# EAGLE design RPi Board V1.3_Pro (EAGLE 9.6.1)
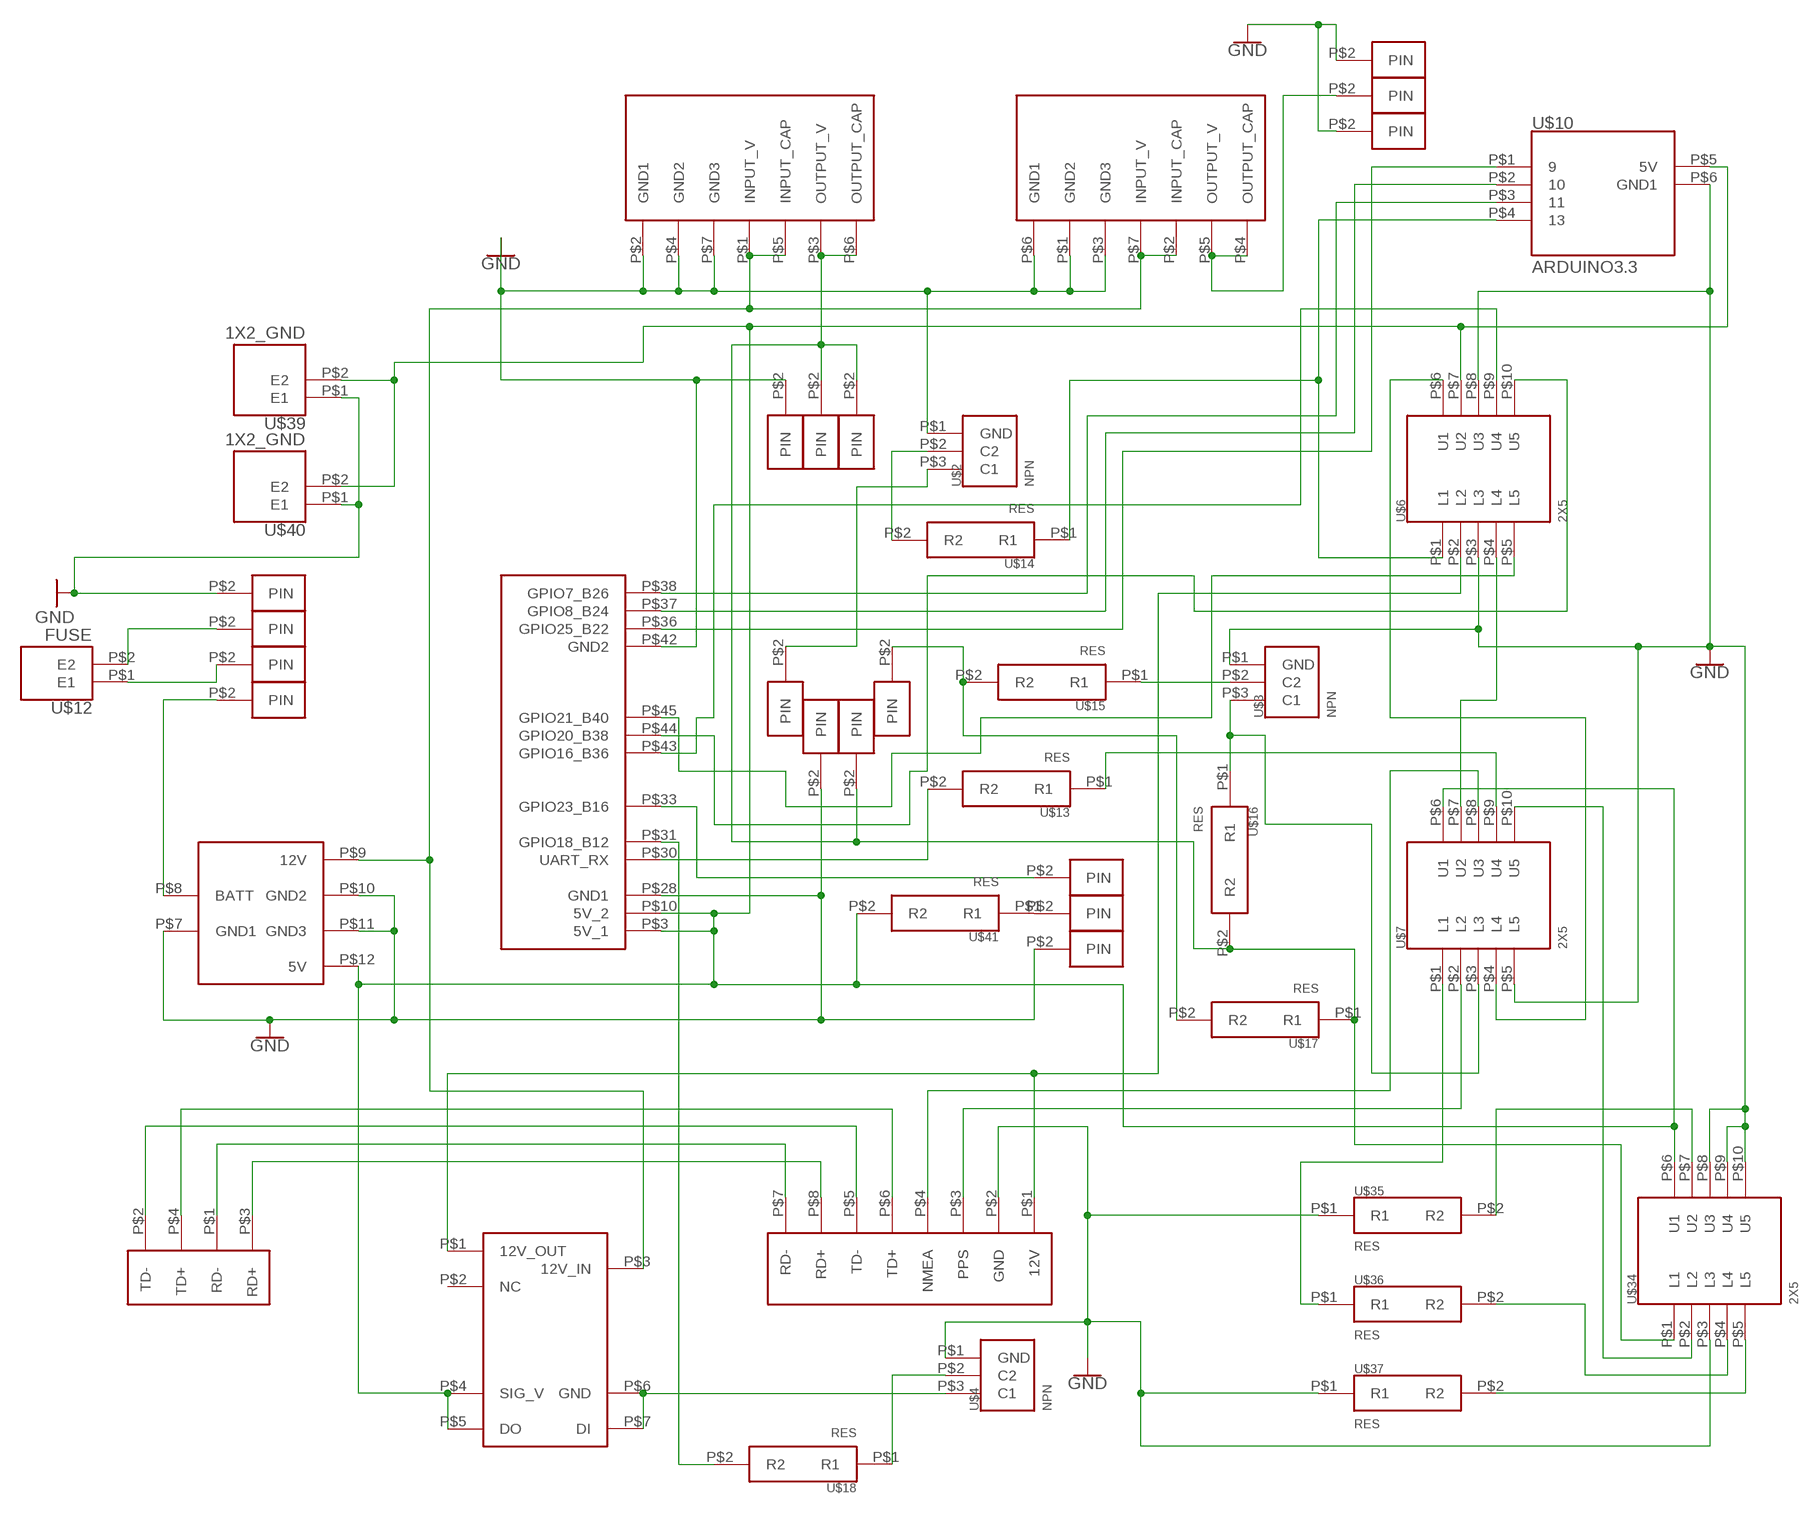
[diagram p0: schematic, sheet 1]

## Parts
U$1  RPI_1X20  [F_RPI_1X20]
U$2  NPN  [F_NPN]
U$3  NPN  [F_NPN]
U$4  NPN  [F_NPN]
U$5  LIDAR  [F_LIDAR]
U$6  2X5  [F_2X5]
U$7  2X5  [F_2X5]
U$8  3.3V_REG  [F_3.3V_REG]
U$9  9V_REG  [F_9V_REG]
U$10  ARDUINO3.3  [F_ARDUINO3.3]
U$11  ETH  [F_ETH]
U$12  FUSE  [F_FUSE]
U$13  RES  [F_RES]
U$14  RES  [F_RES]
U$15  RES  [F_RES]
U$16  RES  [F_RES]
U$17  RES  [F_RES]
U$18  RES  [F_RES]
U$19  1X1  [F_1X1]
U$20  1X1  [F_1X1]
U$21  1X1  [F_1X1]
U$22  1X1  [F_1X1]
U$23  12V_5V_REG  [F_12V_5V_REG]
U$24  1X1  [F_1X1]
U$25  RELAY  [F_RELAY]
U$26  1X1  [F_1X1]
U$27  1X1  [F_1X1]
U$28  1X1  [F_1X1]
U$29  1X1  [F_1X1]
U$30  1X1  [F_1X1]
U$31  1X1  [F_1X1]
U$32  1X1  [F_1X1]
U$33  1X1  [F_1X1]
U$34  2X5  [F_2X5]
U$35  RES  [F_RES]
U$36  RES  [F_RES]
U$37  RES  [F_RES]
U$38  1X1  [F_1X1]
U$39  1X2_GND  [F_1X2_GND]
U$40  1X2_GND  [F_1X2_GND]
U$41  RES  [F_RES]
U$42  1X1  [F_1X1]
U$43  1X1  [F_1X1]
U$44  1X1  [F_1X1]

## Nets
GND: U$1.P$28(GND1) U$1.P$42(GND2) U$2.P$1(GND) U$3.P$1(GND) U$4.P$1(GND) U$5.P$2(GND) U$6.P$3(L3) U$6.P$8(U3) U$7.P$5(L5) U$8.P$2(GND1) U$8.P$4(GND2) U$8.P$7(GND3) U$9.P$1(GND2) U$9.P$3(GND3) U$9.P$6(GND1) U$10.P$6(GND1) U$22.P$2(PIN) U$23.P$7(GND1) U$23.P$10(GND2) U$23.P$11(GND3) U$26.P$2(PIN) U$28.P$2(PIN) U$30.P$2(PIN) U$34.P$3(L3) U$34.P$8(U3) U$34.P$9(U4) U$34.P$10(U5) U$35.P$1(R1) U$37.P$1(R1) U$39.P$1(E1) U$40.P$1(E1) U$43.P$2(PIN) U$44.P$2(PIN)
N$1: U$12.P$2(E2) U$19.P$2(PIN)
N$2: U$12.P$1(E1) U$20.P$2(PIN)
N$3: U$21.P$2(PIN) U$23.P$8(BATT)
N$4: U$5.P$7(RD-) U$11.P$1(RD-)
N$5: U$5.P$8(RD+) U$11.P$3(RD+)
N$6: U$5.P$5(TD-) U$11.P$2(TD-)
N$7: U$41.P$1(R1) U$42.P$2(PIN)
N$8: U$8.P$3(OUTPUT_V) U$8.P$6(OUTPUT_CAP) U$16.P$2(R2) U$17.P$1(R1) U$24.P$2(PIN) U$27.P$2(PIN) U$32.P$2(PIN) U$34.P$1(L1)
N$9: U$5.P$6(TD+) U$11.P$4(TD+)
N$10: U$5.P$3(PPS) U$7.P$2(L2)
N$11: U$7.P$9(U4) U$13.P$1(R1)
N$12: U$1.P$30(UART_RX) U$13.P$2(R2)
N$13: U$5.P$1(12V) U$6.P$2(L2) U$25.P$1(12V_OUT)
N$14: U$6.P$6(U1) U$7.P$4(L4)
N$15: U$6.P$4(L4) U$7.P$7(U2)
N$16: U$1.P$3(5V_1) U$1.P$10(5V_2) U$6.P$7(U2) U$7.P$6(U1) U$10.P$5(5V) U$23.P$12(5V) U$25.P$4(SIG_V) U$25.P$5(DO) U$34.P$6(U1) U$39.P$2(E2) U$40.P$2(E2) U$41.P$2(R2)
N$17: U$5.P$4(NMEA) U$7.P$8(U3)
N$19: U$1.P$36(GPIO25_B22) U$10.P$1
N$20: U$1.P$37(GPIO8_B24) U$10.P$2
N$21: U$8.P$1(INPUT_V) U$8.P$5(INPUT_CAP) U$9.P$2(INPUT_CAP) U$9.P$7(INPUT_V) U$23.P$9(12V) U$25.P$3(12V_IN)
N$22: U$1.P$38(GPIO7_B26) U$10.P$3
N$23: U$9.P$4(OUTPUT_CAP) U$9.P$5(OUTPUT_V) U$29.P$2(PIN)
N$24: U$2.P$2(C2) U$14.P$2(R2)
N$25: U$6.P$1(L1) U$10.P$4 U$14.P$1(R1)
N$26: U$2.P$3(C1) U$31.P$2(PIN)
N$27: U$15.P$2(R2) U$17.P$2(R2) U$33.P$2(PIN)
N$28: U$3.P$2(C2) U$15.P$1(R1)
N$29: U$3.P$3(C1) U$7.P$3(L3) U$16.P$1(R1)
N$30: U$4.P$3(C1) U$25.P$6(GND) U$25.P$7(DI)
N$31: U$4.P$2(C2) U$18.P$1(R1)
N$32: U$1.P$44(GPIO20_B38) U$6.P$10(U5)
N$33: U$1.P$31(GPIO18_B12) U$18.P$2(R2)
N$34: U$1.P$43(GPIO16_B36) U$6.P$9(U4)
N$35: U$7.P$10(U5) U$34.P$2(L2)
N$36: U$34.P$7(U2) U$35.P$2(R2)
N$37: U$1.P$33(GPIO23_B16) U$38.P$2(PIN)
N$38: U$34.P$5(L5) U$37.P$2(R2)
N$39: U$34.P$4(L4) U$36.P$2(R2)
N$40: U$7.P$1(L1) U$36.P$1(R1)
N$42: U$1.P$45(GPIO21_B40) U$6.P$5(L5)
Unconnected: U$25.P$2(NC)

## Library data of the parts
U$1 = OpenMMS_Production:RPI_1X20
U$2-U$4 = OpenMMS_Production:NPN
U$5 = OpenMMS_Production:LIDAR
U$6 U$7 U$34 = OpenMMS_Production:2X5
U$8 = OpenMMS_Production:3.3V_REG
U$9 = OpenMMS_Production:9V_REG
U$10 = OpenMMS_Production:ARDUINO3.3
U$11 = OpenMMS_Production:ETH
U$12 = OpenMMS_Production:FUSE
U$13-U$18 U$35-U$37 U$41 = OpenMMS_Production:RES
U$19-U$22 U$24 U$26-U$33 U$38 U$42-U$44 = OpenMMS_Production:1X1
U$23 = OpenMMS_Production:12V_5V_REG
U$25 = OpenMMS_Production:RELAY
U$39 U$40 = OpenMMS_Production:1X2_GND

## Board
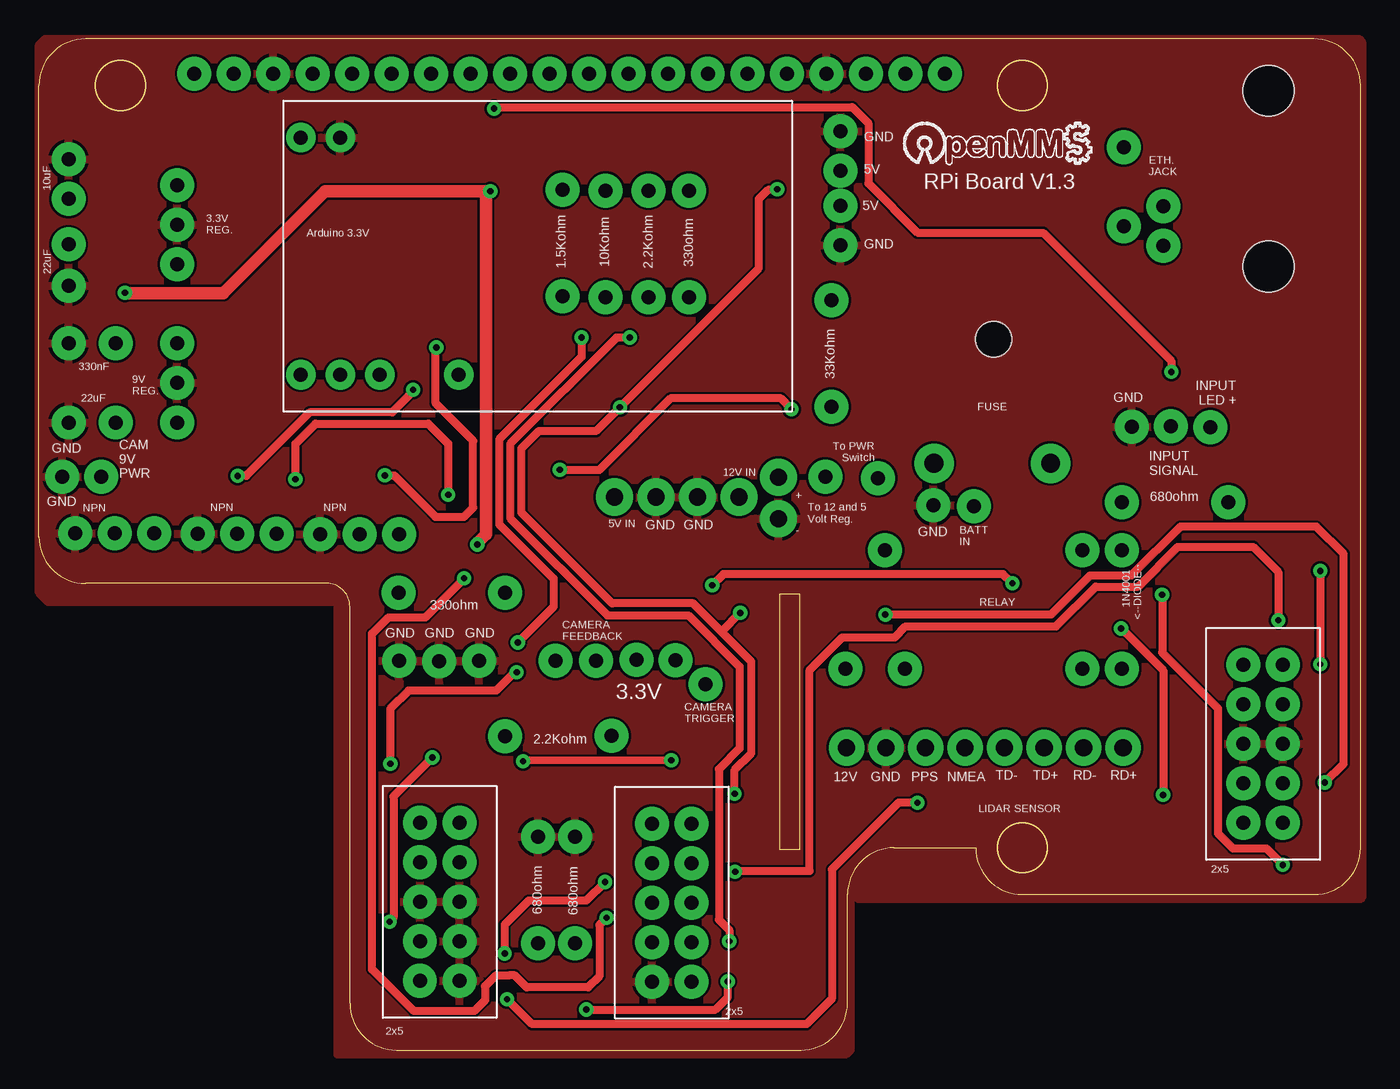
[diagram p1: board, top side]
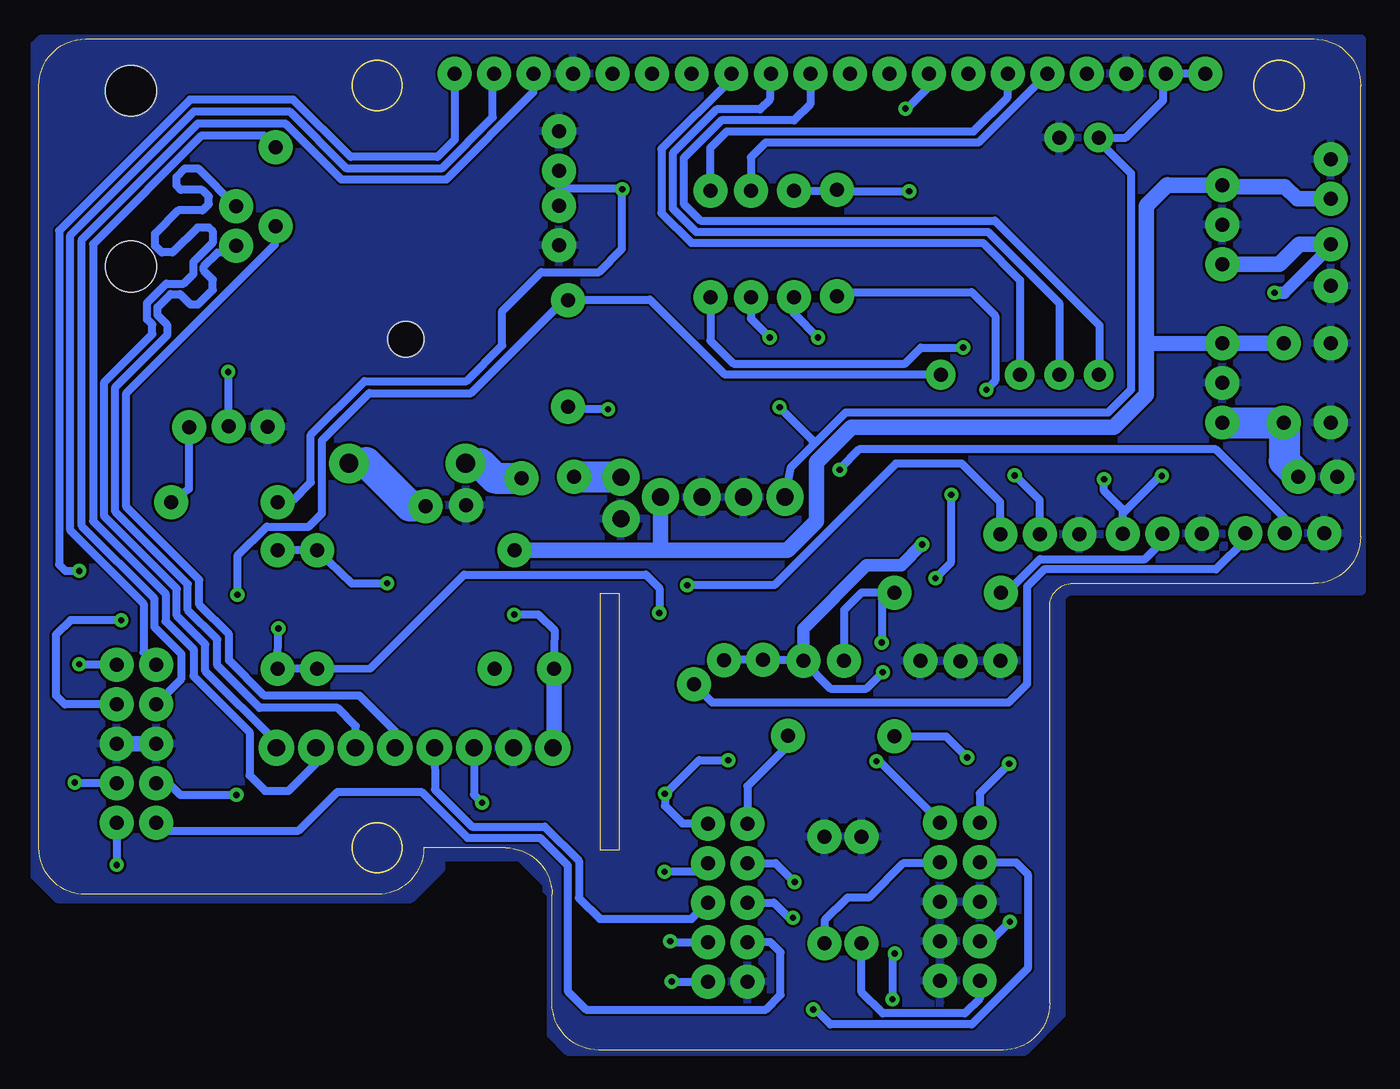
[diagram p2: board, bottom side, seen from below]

Size 85 x 65 mm. Coordinates in mm from the lower left corner, seen from the top.
Outline: 48.9,12.86 47.65,12.86 47.65,29.32 48.9,29.32 48.9,12.86
Outline: 20,3 arc90 23,0 49,0 arc90 52,3 52,10 arc-90 55,13 60.25,13 arc90 63.25,10 82,10 arc90 85,13 85,62 arc90 82,65 3,65 arc90 0,62 0,33 arc90 3,30 18.5,30 arc-90 20,28.5 20,3
Outline: circle at 63.25,62 radius 1.6
Outline: circle at 63.25,13 radius 1.6
Outline: circle at 5.25,62 radius 1.6
Copper layers (1*16): Top 0.035mm / dielectric 1.5mm / Bottom 0.035mm
Design rules "OpenMMS_Production": minimum track width 20mil, minimum drill 0.4mm, track to track 6mil, track to pad 6mil, pad to pad 6mil, via to via 6mil, smd to smd 6mil, copper to edge 0mil, drill to drill 0mil, minimum pad ring 10mil, minimum via ring 10mil, stop-mask expansion 4mil, vias tented up to drill 0mil, thermal gap 8mil

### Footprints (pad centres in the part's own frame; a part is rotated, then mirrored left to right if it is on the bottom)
F_RPI_1X20 = drill 0.9 pad 2.184: P$3 0,0; P$10 2.54,0; P$28 5.08,0; P$29 7.62,0; P$30 10.16,0; P$31 12.7,0; P$32 15.24,0; P$33 17.78,0; P$34 20.32,0; P$35 22.86,0; P$36 25.4,0; P$37 27.94,0; P$38 30.48,0; P$39 33.02,0; P$40 35.56,0; P$41 38.1,0; P$42 40.64,0; P$43 43.18,0; P$44 45.72,0; P$45 48.26,0
F_NPN = drill 0.9 pad 2.184: P$1 2.54,0; P$2 0,0; P$3 -2.54,0
F_LIDAR = drill 1.1 pad 2.3: P$1 -9.017,-0.254; P$2 -6.477,-0.254; P$3 -3.937,-0.254; P$4 -1.397,-0.254; P$5 1.143,-0.254; P$6 3.683,-0.254; P$7 6.223,-0.254; P$8 8.763,-0.254
F_2X5 = drill 0.9 pad 2.184: P$1 -5.08,-1.27; P$2 -2.54,-1.27; P$3 0,-1.27; P$4 2.54,-1.27; P$5 5.08,-1.27; P$6 -5.08,1.27; P$7 -2.54,1.27; P$8 0,1.27; P$9 2.54,1.27; P$10 5.08,1.27
F_3.3V_REG = drill 0.9 pad 2.184: P$1 3.175,1.905; P$2 3.175,-0.635; P$3 3.175,-3.175; P$4 -3.81,3.556; P$5 -3.81,1.016; P$6 -3.81,-1.905; P$7 -3.81,-4.572
F_9V_REG = drill 0.9 pad 2.184: P$1 -3.81,2.032; P$2 -0.762,2.032; P$3 -3.81,-3.048; P$4 -0.762,-3.048; P$5 3.175,-3.048; P$6 3.175,-0.508; P$7 3.175,2.032
F_ARDUINO3.3 = drill 0.9 pad 1.9: P$1 -7.62,13.97; P$2 -7.62,11.43; P$3 -7.62,8.89; P$4 -7.62,3.81; P$5 7.62,13.97; P$6 7.62,11.43
F_ETH = drill 0.9 pad 2.184: P$1 -5.842,2.159; P$2 -5.842,-2.921; P$3 -3.302,-1.651; P$4 -3.302,-4.191 | hole 3.25: 3.47,5.79; 3.47,-5.51
F_FUSE = drill 1.2 pad 2.54: P$1 -0.508,3.937; P$2 -0.508,-3.556 | hole 2.3: 7.47,0.11
F_RES = drill 0.9 pad 2.184: P$1 0,3.81; P$2 0,-3.048
F_1X1 = drill 0.9 pad 2.184: P$2 0,0
F_12V_5V_REG = drill 1.1 pad 2.4: P$7 -5.08,1.397; P$8 -5.08,-1.27; P$9 -2.54,0; P$10 0.127,0; P$11 2.794,0; P$12 5.461,0
F_RELAY = drill 0.9 pad 2.184: P$1 -3.81,8.89; P$2 -3.81,5.08; P$3 3.81,6.35; P$4 -3.81,-6.35; P$5 -3.81,-8.89; P$6 3.81,-6.35; P$7 3.81,-8.89
F_1X2_GND = drill 0.9 pad 2.184: P$1 0,1.27; P$2 0,-1.27

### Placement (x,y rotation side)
U$1  9.99,62.77 0 top
U$2  4.89,33.22 180 top
U$3  12.74,33.19 180 top
U$4  20.64,33.15 180 top
U$5  60.96,19.68 0 top
U$6  78.74,19.68 90 top
U$7  40.7,9.47 270 top
U$8  5.72,53.7 0 top
U$9  5.72,43.39 0 top
U$10  30.81,51.03 90 top
U$11  75.61,55.88 0 top
U$12  61.5,38.23 90 top
U$13  39.21,52.2 180 top
U$14  50.97,44.4 0 top
U$15  26.93,29.4 90 top
U$16  33.66,52.25 180 top
U$17  36.45,51.44 0 top
U$18  41.81,52.2 180 top
U$19  60.12,34.97 0 top
U$20  53.97,36.76 270 top
U$21  50.57,36.85 0 top
U$22  57.53,35.01 0 top
U$23  42.48,35.55 180 top
U$24  40.93,25.05 270 top
U$25  60.76,28.31 90 top
U$26  23.16,25.02 90 top
U$27  38.42,25.09 90 top
U$28  25.74,24.99 90 top
U$29  4.01,36.86 180 top
U$30  28.3,25.02 90 top
U$31  42.87,23.51 90 top
U$32  35.84,25.02 90 top
U$33  33.22,25.02 90 top
U$34  25.77,9.53 270 top
U$35  34.47,9.9 0 top
U$36  33.03,20.17 270.3 top
U$37  32.09,9.9 0 top
U$38  72.8,40.1 90 top
U$39  51.56,57.79 0 top
U$40  51.56,52.99 180 top
U$41  72.69,35.22 270 top
U$42  75.34,40.03 90 top
U$43  70.29,40.06 90 top
U$44  1.5,36.86 0 top

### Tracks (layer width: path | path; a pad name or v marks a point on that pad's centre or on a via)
GND
  Bottom 1: U$6.P$8 U$6.P$3
  pour Bottom: -0.1,65 84.9,65 85.3,64.6 85.3,11.2 83.8,9.7 61.1,9.7 59.1,11.7 59.1,12.5 59,12.4 54.1,12.4 52.4,10.7 52.4,10.3 52.1,10 52.1,1 51,-0.1 21.6,-0.1 19.2,2.3 19.2,29.1 18.8,29.5 -0.1,29.5
  pour Top: 0.4,65 84.9,65 85.1,64.8 85.1,9.8 85,9.7 52.7,9.7 52.2,10.2 52.2,0 51.9,-0.3 19.2,-0.3 19.2,28.4 19.6,28.8 0.6,28.8 0,29.4 0,64.6
N$1
  Bottom 0.508: U$12.P$2 65.06,37.76
  Bottom 2: 65.06,37.76 63.93,37.76 61.14,34.97 U$19.P$2
N$2
  Bottom 2: U$12.P$1 56.63,37.72 55.67,36.76 U$20.P$2
N$3
  Bottom 2: U$21.P$2 47.59,36.85 U$23.P$8
N$4
  Bottom 0.508: U$5.P$7 67.17,18.43 68.95,16.65 70.45,16.65 71.46,17.66 71.46,20.44 75.06,24.04 75.06,25.77 76.85,27.55 76.85,29.33 81.52,34 81.52,51.8 74.52,58.8 70.53,58.8 U$11.P$1
N$5
  Bottom 0.508: U$5.P$8 69.72,19.78 74.3,24.35 74.3,26.08 76.13,27.92 76.13,29.65 80.79,34.31 80.79,42.93 77.7,46.02 77.7,46.64 78.03,46.98 78.03,48.02 76.8,49.26 75.69,49.26 75.06,49.89 75.06,50.67 73.8,51.93 73.8,52.6 74.08,52.88 74.8,52.88 76.4,51.27 77.1,51.27 77.53,51.7 77.53,52.48 76.03,53.98 74.47,53.98 74.08,54.38 74.08,54.88 74.5,55.3 75.88,55.3 76.15,55.58 76.15,56.11 75.59,56.67 74.77,56.67 72.33,54.23 U$11.P$3
N$6
  Bottom 0.508: U$5.P$5 62.07,20.47 64.38,22.78 70.51,22.78 72.77,25.04 72.77,26.71 74.69,28.63 74.69,30.23 79.37,34.91 79.37,42.23 69.82,51.79 U$11.P$2
N$7
  Bottom 0.508: U$41.P$1 75.34,36.07 U$42.P$2
N$8  (via drill 0.4)
  Top 0.508: v5.53,48.68 5.56,48.65 | v28.2,32.5 28.2,32.6 | 28.76,54.93 v29.03,55.2 | v30.73,24.28 30.58,24.28 29.41,23.1 23.77,23.1 22.6,21.93 v22.6,18.4
  Top 0.8: 5.56,48.65 11.86,48.65 18.41,55.2 v29.03,55.2 | 28.2,32.6 28.76,33.16 28.76,54.93
  Bottom 0.508: v29.03,55.2 32.63,55.2 U$16.P$2 | U$17.P$1 33.72,55.25 | U$27.P$2 35.92,25.09 | v30.73,24.28 31.78,23.23 34.09,23.23 35.84,24.98 U$32.P$2 | v22.6,18.4 24.5,16.5 U$34.P$1 | U$27.P$2 40.89,25.09 U$24.P$2 | 8.83,50.5 U$8.P$3
  Bottom 0.8: v28.2,32.5 29.55,31.15 31.77,31.15 35.84,27.08 U$32.P$2 | U$8.P$6 1.91,51.68 4.91,48.68 v5.53,48.68
  Bottom 1: U$8.P$6 3.93,51.79 5.22,50.5 8.83,50.5
  Bottom 2: U$16.P$2 33.72,55.25 | U$27.P$2 | U$32.P$2 35.92,25.09
N$9
  Bottom 0.508: U$5.P$6 64.62,20.82 65.8,22 70.8,22 73.53,24.73 73.53,26.4 75.42,28.29 75.42,29.95 80.08,34.61 80.08,42.61 76.75,45.94 76.75,46.62 77.38,47.25 77.38,47.75 76.53,48.6 75.92,48.6 75.26,47.93 74.76,47.93 73.82,48.87 73.82,49.52 74.4,50.1 74.4,50.38 73.51,51.27 72.67,51.32 U$11.P$4
N$10  (via drill 0.4)
  Top 0.508: v36.4,10.8 35.2,9.6 31.5,9.6 29.96,8.06 v29.96,6.2 | v30.12,3.27 31.72,1.67 49.37,1.67 50.99,3.29 50.99,11.61 55.28,15.9 v56.5,15.9
  Bottom 0.508: U$7.P$2 37.62,12.02 v36.4,10.8 | v29.96,6.2 30.12,6.05 v30.12,3.27 | U$5.P$3 57.02,16.42 v56.5,15.9
N$11  (via drill 0.4)
  Top 0.508: v38,45.8 37.15,45.8 30.31,38.97 30.31,34.19 36.56,27.94 41.76,27.94 45.06,24.65 45.06,19.4 43.73,18.06 43.73,8.38 44.4,7.7 v44.4,7
  Bottom 0.508: U$13.P$1 39.21,47.01 v38,45.8 | v44.4,7 44.34,6.93 U$7.P$9
N$12
  Bottom 0.508: U$1.P$30 24.6,58.33 38.27,58.33 39.21,57.39 U$13.P$2
N$13  (via drill 0.4)
  Top 0.508: v82.7,17.2 83.9,18.4 83.9,31.9 82.15,33.65 73.42,33.65 70.27,30.5 67.6,30.5 65.09,27.99 v54.43,27.99
  Bottom 0.508: U$25.P$1 51.82,26.94 52.87,27.99 v54.43,27.99 | U$6.P$2 82.64,17.14 v82.7,17.2 | 51.87,19.5 U$5.P$1
  Bottom 1: U$25.P$1 51.87,19.5
N$14
  Bottom 0.508: U$7.P$4 37.96,6.93 37.3,6.28 37.3,3.55 38.25,2.6 49.8,2.6 50.99,3.79 50.99,11.87 52.76,13.64 57.44,13.64 60.4,16.6 65.8,16.6 68.3,14.1 76.97,14.1 U$6.P$6
N$15  (via drill 0.4)
  Top 0.508: v44.77,11.45 44.83,11.5 49.56,11.5 49.56,24.41 51.67,26.52 55.04,26.52 55.74,27.23 65.41,27.23 67.97,29.79 70.7,29.79 73.24,32.34 78.1,32.34 79.7,30.73 v79.7,27.63
  Bottom 0.508: v79.7,27.63 82.97,27.63 83.9,26.7 83.9,22.8 83.33,22.23 U$6.P$4 | U$7.P$7 41.98,11.45 v44.77,11.45
N$16  (via drill 0.4)
  Top 0.508: v44.74,16.48 44.74,18 45.82,19.08 45.82,24.96 43.89,26.89 | 43.89,26.89 42.08,28.7 36.87,28.7 31.03,34.55 31.03,38.67 32.14,39.79 35.82,39.79 v37.36,41.32 46.31,50.27 46.31,54.71 46.89,55.29 47.44,55.29 v47.48,55.34 | v45.1,28.1 43.89,26.89 | v69.6,27.1 72.3,24.4 v72.3,16.4 | v40.66,18.63 31.17,18.6 v31.13,18.56
  Bottom 0.508: U$1.P$3 U$1.P$10 12.7,62.61 12.7,61.05 15.11,58.65 U$10.P$5 16.84,58.42 14.76,56.34 14.76,42.47 16.23,41 33.1,41 35.25,38.85 | 35.25,38.85 36.64,37.46 U$23.P$12 | U$34.P$6 27.71,15.27 27.71,15.3 30.96,18.56 v31.13,18.56 | v37.36,41.32 35.25,39.21 35.25,38.85 | v40.66,18.63 42.54,18.63 44.69,16.48 v44.74,16.48 44.74,15.69 43.62,14.57 41.99,14.57 U$7.P$6 | v45.1,28.1 45.1,29.7 45.96,30.56 57.65,30.56 63.67,24.54 U$25.P$4 U$25.P$5 69.62,27.08 v69.6,27.1 | v72.3,16.4 75.9,16.4 76.64,17.14 U$6.P$7 | U$41.P$2 69.26,35.22 69.13,35.34 68.66,35.34 67.51,36.49 67.51,39.55 64.06,43 57.51,43 55.21,45.3 55.21,47.49 52.69,50.01 48.99,50.01 47.5,51.5 47.5,55.31 v47.48,55.34 47.53,55.39 51.46,55.39 51.56,55.49 U$39.P$2 U$40.P$2
N$17
  Bottom 0.508: U$7.P$8 43.02,8.43 48.92,8.43 50.27,9.77 50.27,12.16 52.47,14.36 57.15,14.36 59.53,16.74 U$5.P$4
N$19
  Bottom 0.508: U$1.P$36 35.4,60.8 36.44,59.76 41.12,59.76 43.54,57.34 43.54,54.4 42.45,53.31 23.52,53.31 16.8,46.59 16.8,43.45 U$10.P$1
N$20
  Bottom 0.508: U$1.P$37 38,62.71 38,61.1 38.63,60.47 41.41,60.47 44.25,57.64 44.25,54.11 42.74,52.6 23.96,52.6 19.38,48.02 U$10.P$2
N$21
  Bottom 0.508: 8.77,55.5 U$8.P$1 | U$25.P$3 | 12.42,55.6 12.45,55.63
  Bottom 1: 8.77,55.5 4.87,55.5 4.08,54.71 U$8.P$5 | U$9.P$2 U$9.P$7 13.78,45.42 | 13.78,45.42 13.78,42.11 15.86,40.03 32.74,40.03 34.98,37.79 34.98,33.99 36.86,32.11 42.9,32.11 45.02,32.11 | 45.02,32.11 U$25.P$3 | 13.78,45.42 13.78,54.29 12.45,55.63 | U$8.P$1 12.42,55.6 | U$23.P$9 45.02,32.11
N$22
  Bottom 0.508: U$1.P$38 40.48,62.42 44.96,57.93 44.96,53.8 43.04,51.89 24.29,51.89 21.9,49.5 21.92,49.48 U$10.P$3
N$23
  Bottom 0.508: U$9.P$4 4.91,40.3 | U$29.P$2 3.96,36.91
  Bottom 2: U$9.P$5 U$9.P$4 | 4.91,40.3 4.91,37.86 3.96,36.91
N$24  (via drill 0.4)
  Top 0.508: v33.5,37.3 36.04,37.3 40.63,41.89 47.71,41.89 v48.4,41.2
  Bottom 0.508: U$2.P$2 4.89,34.19 9.32,38.62 32.25,38.62 33.5,37.37 v33.5,37.3 | U$14.P$2 50.67,41.2 v48.4,41.2
N$25  (via drill 0.4)
  Top 0.508: v72.23,29.27 72.23,25.54 75.82,21.96 75.82,13.92 76.79,12.95 78.95,12.95 v80,11.9
  Bottom 0.508: U$10.P$4 40.87,43.41 45.7,48.24 50.94,48.24 U$14.P$1 51.22,48.21 57.21,42.23 63.75,42.23 66.8,39.18 66.8,34.5 67.65,33.65 70.35,33.65 72.23,31.76 v72.23,29.27 | U$6.P$1 v80.01,11.91 v80,11.9
N$26
  Bottom 0.508: U$2.P$3 7.43,32.77 9.31,30.89 20.34,30.89 21.45,29.78 21.45,23.52 22.65,22.33 41.68,22.33 U$31.P$2
N$27  (via drill 0.4)
  Top 0.508: v34.9,45.8 34.9,44.56 29.6,39.26 29.6,33.8 33.1,30.3 33.1,28.5 v30.8,26.2
  Bottom 0.508: U$33.P$2 33.23,28.27 32.1,29.4 U$15.P$2 30.8,29.03 v30.8,26.2 | U$17.P$2 36.45,47.35 v34.9,45.8
N$28
  Bottom 0.508: U$3.P$2 12.74,32.69 13.87,31.55 20.62,31.55 22.78,29.4 U$15.P$1
N$29  (via drill 0.4)
  Top 0.508: v24.07,42.45 24.07,42.34 22.72,41 17.42,41 13.34,36.91 v12.79,36.91 | v16.5,36.7 16.5,38.98 17.79,40.27 25.04,40.27 26.33,38.99 v26.33,35.7 | v27.34,30.33 27.34,30.29 24.87,27.81 22.48,27.81 21.43,26.76 21.43,5.18 24.12,2.49 27.99,2.49 28.7,3.2 28.69,3.21 28.69,4.1 29.38,4.79 30.21,4.79 30.22,4.8 30.6,4.8 31.37,4.03 35.32,4.03 36.04,4.75 36.04,8.04 v36.5,8.5
  Bottom 0.508: U$16.P$1 33.39,48.71 25.01,48.71 23.5,47.2 23.5,43.02 v24.07,42.45 | v12.79,36.91 12.89,36.91 15.28,34.52 U$3.P$3 15.28,34.72 16.5,35.94 v16.5,36.7 | v26.33,35.7 26.36,35.67 26.36,31.31 v27.34,30.33 | v36.5,8.5 36.75,8.5 37.73,9.47 U$7.P$3
N$30  (via drill 0.4)
  Top 0.508: v43.3,29.88 44.02,30.6 62,30.6 v62.6,30
  Bottom 0.508: U$4.P$3 23.18,35.22 25.65,37.7 29.89,37.7 37.7,29.88 v43.3,29.88 | v62.6,30 64.88,30 U$25.P$6 U$25.P$7
N$31  (via drill 0.4)
  Top 0.508: v25.56,45.16 25.52,45.12 25.52,41.57 27.92,39.16 27.92,34.86 27.34,34.28 25.51,34.28 22.85,36.94 v22.25,36.94
  Bottom 0.508: U$18.P$1 41.81,45.61 40.33,44.13 29.3,44.13 28.29,45.15 25.58,45.15 v25.56,45.16 | U$4.P$2 20.64,35.34 22.24,36.95 v22.25,36.94
N$32
  Bottom 0.508: U$1.P$44 55.81,62.67 55.81,59.95 59.06,56.7 65.25,56.7 68.89,60.34 75.02,60.34 82.97,52.39 82.97,33.4 78.27,28.7 78.27,25.57 U$6.P$10
N$33
  Bottom 0.508: U$1.P$31 22.7,61.25 24.9,59.05 40.75,59.05 41.81,57.99 U$18.P$2
N$34
  Bottom 0.508: U$1.P$43 53.2,62.74 53.2,61.56 58.79,55.98 65.55,55.98 69.15,59.57 74.76,59.57 82.24,52.1 82.24,33.69 77.56,29.01 77.56,27.19 75.82,25.45 75.82,23.88 U$6.P$9
N$35  (via drill 0.4)
  Top 0.508: v35.2,2.6 43.5,2.6 44.3,3.4 v44.3,4.4
  Bottom 0.508: U$34.P$2 22.16,12.06 21.41,11.31 21.41,5.25 25.01,1.65 34.1,1.65 34.98,2.52 35.12,2.52 v35.2,2.6 | v44.3,4.4 v44.3,4.39 U$7.P$10
N$36
  Bottom 0.508: U$34.P$7 27.11,12 29.42,12 31.62,9.8 33,9.8 34.47,8.33 U$35.P$2
N$37  (via drill 0.4)
  Top 0.508: v72.82,43.59 72.82,44.3 64.59,52.52 60.8,52.52 56.5,52.55 53.34,55.71 53.34,59.59 52.31,60.61 29.36,60.61 v29.27,60.52
  Bottom 0.508: U$1.P$33 27.77,61.92 29.18,60.52 v29.27,60.52 | U$38.P$2 72.82,40.12 v72.82,43.59
N$38
  Bottom 0.508: U$34.P$5 24.5,3.3 25.45,2.35 30.73,2.35 32.1,3.73 32.1,6.39 U$37.P$2
N$39  (via drill 0.4)
  Top 0.508: v22.55,8.24 22.8,8.49 22.8,16.3 v25.3,18.8
  Bottom 0.508: U$34.P$4 23.8,6.99 v22.55,8.24 | v25.3,18.8 26.65,20.15 U$36.P$2
N$40
  Bottom 0.508: U$7.P$1 39.44,16.96 36.84,19.56 U$36.P$1
N$42  (via drill 0.4)
  Top 0.508: v82.4,30.8 v82.4,24.8
  Bottom 0.508: U$1.P$45 58.26,58.52 59.36,57.41 64.95,57.41 68.64,61.1 75.27,61.1 83.7,52.67 83.7,31.2 83.3,30.8 v82.4,30.8 | U$6.P$5 82.36,24.77 v82.4,24.8

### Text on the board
tPlace: GND | 5V | ETH. / JACK | 10uF | RPi Board V1.3 | 5V | 3.3V / REG. | Arduino 3.3V | GND | 22uF | 1.5Kohm | 10Kohm | 2.2Kohm | 330ohm | 330nF | 33Kohm | INPUT / LED + | 22uF | 9V / REG. | GND | FUSE | GND | To PWR / Switch | CAM / 9V / PWR | 12V IN | INPUT / SIGNAL | GND | NPN | NPN | NPN | 680ohm | 5V IN | GND | GND | GND | + / To 12 and 5 / Volt Reg. / - | BATT / IN | 330ohm | RELAY | 1N4001 / <--DIODE-- | GND | GND | GND | CAMERA / FEEDBACK | 3.3V | CAMERA / TRIGGER | 2.2Kohm | 12V | GND | PPS | NMEA | TD- | TD+ | RD- | RD+ | LIDAR SENSOR | 2x5 | 680ohm | 680ohm | 2x5 | 2x5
